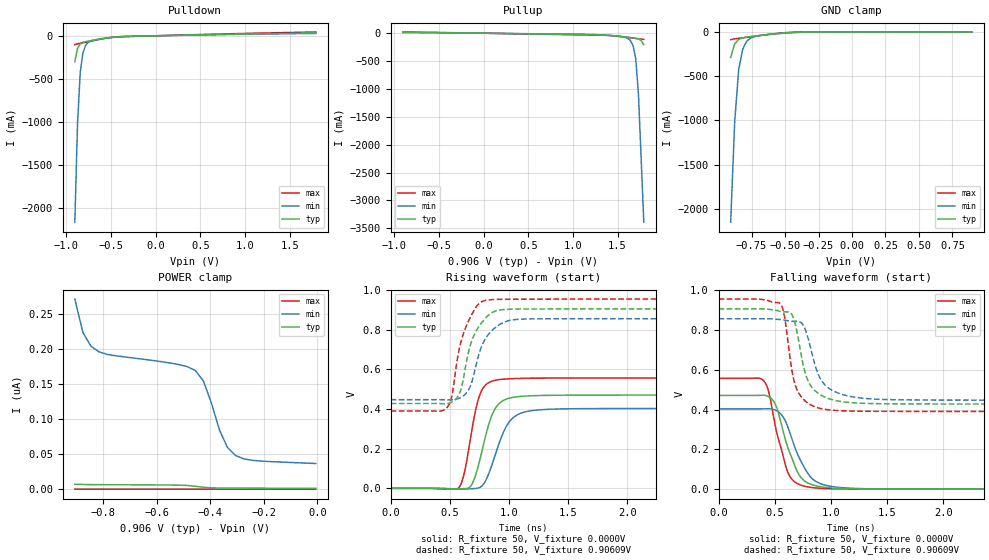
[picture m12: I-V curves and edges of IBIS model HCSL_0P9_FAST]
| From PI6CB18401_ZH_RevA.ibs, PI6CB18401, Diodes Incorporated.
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[Model]   HCSL_0P9_FAST
Model_type Output
Vref=0.9000V
Vmeas=900mV
| variable   typ   min   max
C_comp   2.000pF   1.970pF   2.030pF
[Voltage Range]   0.90609V   0.85650V   0.95550V
[POWER Clamp Reference]   0.90609V   0.85650V   0.95550V
[GND Clamp Reference]   0.0000V   0.0000V   0.0000V
[Pullup Reference]   0.90609V   0.85650V   0.95550V
[Pulldown Reference]   0.0000V   0.0000V   0.0000V
[Temperature Range]   25   85   -40
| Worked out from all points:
|   slope of the pulldown table from 0 to 0.136 V, typ, clamps not added: 43.9 ohm
|   slope of the pullup table from 0 to 0.136 V, typ, clamps not added: 46.1 ohm
|   GND clamp passes 1 mA (typ) near -0.37 V on its own axis
|   falling waveform, R_fixture 50, V_fixture 0.0000V: 20-80 % time 160ps typ, 183ps min, 137ps max; typ from 0.471 V to 0 V
|   rising waveform, R_fixture 50, V_fixture 0.0000V: 20-80 % time 130ps typ, 155ps min, 105ps max; typ from 0 V to 0.471 V
|   falling waveform, R_fixture 50, V_fixture 0.90609V: 20-80 % time 125ps typ, 150ps min, 102ps max; typ from 0.906 V to 0.428 V
|   rising waveform, R_fixture 50, V_fixture 0.90609V: 20-80 % time 134ps typ, 141ps min, 128ps max; typ from 0.428 V to 0.906 V
[GND Clamp]
| Voltage   I(typ)   I(min)   I(max)
-906.1mV  -286.6mA   -2.151A    -85.45mA
-876.1mV  -133.8mA   -1.017A    -76.33mA
-846.1mV  -83.21mA   -420.9mA   -70.35mA
-816.1mV  -64.75mA   -192.1mA   -65.15mA
-786.1mV  -56.15mA   -103mA     -59.83mA
-756.1mV  -50.17mA   -66.66mA   -53.95mA
-726.1mV  -44.73mA   -50.08mA   -47.66mA
-636.1mV  -29.01mA   -29.59mA   -28.7mA
-486.1mV  -8.023mA   -10.08mA   -5.373mA
-366.1mV  -792.8uA   -1.762mA   -189.4uA
893.9mV   1.274nA    37.22nA    5.411pA
[POWER Clamp]
| Voltage   I(typ)   I(min)   I(max)
-906.1mV  7.102nA    272nA      64.05pA
-876.1mV  6.695nA    224.4nA    62.62pA
-846.1mV  6.537nA    204.6nA    61.28pA
-816.1mV  6.464nA    196.5nA    59.94pA
-516.1mV  5.725nA    178.2nA    42.48pA
-456.1mV  4.154nA    169.7nA    33.31pA
-426.1mV  2.718nA    154.9nA    31.21pA
-366.1mV  1.642nA    84.73nA    27.91pA
-336.1mV  1.538nA    59.52nA    26.32pA
-306.1mV  1.492nA    48.22nA    24.74pA
-246.1mV  1.442nA    41.44nA    21.59pA
-6.09mV   1.286nA    36.73nA    8.971pA
[Pulldown]
| Voltage   I(typ)   I(min)   I(max)
-906.1mV  -299.2mA   -2.161A    -102.5mA
-876.1mV  -146.3mA   -1.027A    -93.22mA
-846.1mV  -95.54mA   -430.5mA   -87.06mA
-816.1mV  -76.95mA   -201.7mA   -81.68mA
-786.1mV  -68.2mA    -112.5mA   -76.16mA
-756.1mV  -62.06mA   -75.95mA   -70.08mA
-726.1mV  -56.46mA   -59.25mA   -63.56mA
-636.1mV  -40.19mA   -38.34mA   -43.86mA
-486.1mV  -17.93mA   -17.86mA   -18.7mA
-336.1mV  -7.911mA   -7.047mA   -9.887mA
1.794V    33.19mA    26.85mA    42.72mA
[Pullup]
| Voltage   I(typ)   I(min)   I(max)
-906.1mV  16mA       13.17mA    20.24mA
1.194V    -25.61mA   -22.08mA   -32.46mA
1.494V    -51.42mA   -53.83mA   -51.13mA
1.614V    -72.36mA   -92.15mA   -74.09mA
1.644V    -77.85mA   -130mA     -80.63mA
1.674V    -83.5mA    -222.9mA   -87.26mA
1.704V    -90.18mA   -461.5mA   -93.77mA
1.734V    -101.4mA   -1.083A    -99.9mA
1.764V    -128.3mA   -2.227A    -105.5mA
1.794V    -205.8mA   -3.39A     -110.7mA
[Falling Waveform]
R_fixture = 50
V_fixture = 0.0000V
V_fixture_min = 0.0000V
V_fixture_max = 0.0000V
|   Time   V(typ)   V(min)   V(max)
0s        471mV      403.2mV    557.1mV
410ps     471.8mV    403.8mV    539.1mV
450ps     464.2mV    404.2mV    480.3mV
510ps     420.1mV    396.3mV    303.3mV
620ps     202.9mV    306.6mV    79.53mV
710ps     78.05mV    166.5mV    25.5mV
790ps     32.44mV    82.81mV    11.66mV
920ps     11.09mV    25.02mV    4.041mV
1.24ns    1.451mV    3.33mV     529.2uV
5ns       24.19uV    25.56uV    22.83uV
[Rising Waveform]
R_fixture = 50
V_fixture = 0.0000V
V_fixture_min = 0.0000V
V_fixture_max = 0.0000V
|   Time   V(typ)   V(min)   V(max)
0s        11.18uV    11.83uV    11.3uV
570ps     -3.289mV   -3.914mV   131.2uV
620ps     -1.827mV   -3.693mV   73.13mV
680ps     14.61mV    -2.221mV   271.9mV
750ps     136.3mV    4.079mV    467.2mV
830ps     325.8mV    76.78mV    534.2mV
890ps     409mV      181.3mV    546.4mV
1.02ns    457.6mV    348.2mV    553.5mV
1.24ns    468.3mV    395.4mV    556.2mV
5ns       470.9mV    403.2mV    557.1mV
[Falling Waveform]
R_fixture = 50
V_fixture = 0.90609V
V_fixture_min = 0.85650V
V_fixture_max = 0.95550V
|   Time   V(typ)   V(min)   V(max)
0s        906.1mV    856.5mV    955.5mV
550ps     893.2mV    852.1mV    932.6mV
590ps     891.4mV    849.2mV    855.8mV
640ps     886mV      844.5mV    642.5mV
690ps     811.3mV    843.8mV    510.5mV
790ps     552.5mV    771.5mV    434.7mV
870ps     488.9mV    602.7mV    411.5mV
930ps     467.1mV    535mV      403mV
1.42ns    429.8mV    451.9mV    391.2mV
5ns       428.3mV    447.7mV    390.8mV
[Rising Waveform]
R_fixture = 50
V_fixture = 0.90609V
V_fixture_min = 0.85650V
V_fixture_max = 0.95550V
|   Time   V(typ)   V(min)   V(max)
0s        428.3mV    447.6mV    390.8mV
480ps     428.5mV    446.8mV    410.9mV
520ps     436.8mV    446.9mV    473.7mV
570ps     466.5mV    453mV      676.4mV
620ps     573.2mV    470mV      790.2mV
690ps     752.8mV    545.2mV    883.4mV
810ps     864.7mV    764.4mV    949.9mV
940ps     901.7mV    833.5mV    954.2mV
1.12ns    905.2mV    854.5mV    954.9mV
5ns       906.1mV    856.5mV    955.5mV
[Ramp]
| variable   typ   min   max
dV/dt_r   0.28315V/129.35p   0.24235V/154.48p   0.33443V/104.88p
dV/dt_f   0.28639V/125.31p   0.24562V/150.05p   0.33866V/101.38p
R_load = 50
